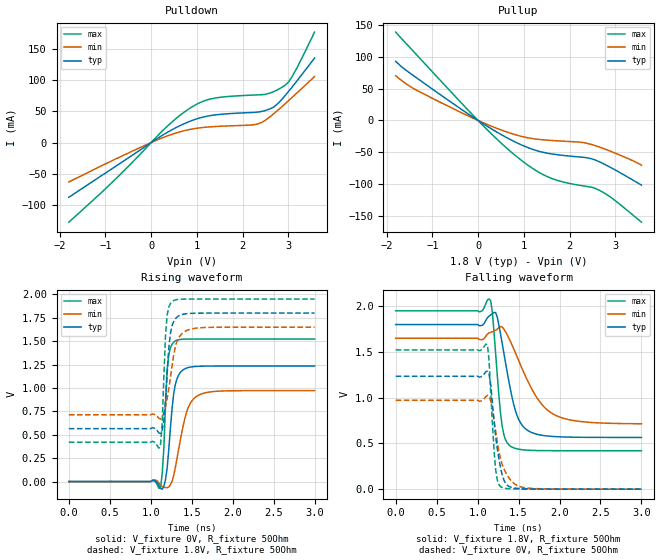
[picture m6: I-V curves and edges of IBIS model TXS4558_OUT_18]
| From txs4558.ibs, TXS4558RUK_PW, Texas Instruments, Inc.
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[Model]   TXS4558_OUT_18
Model_type  Output
Vref =   0
Rref =   50
Cref =   1p
Vmeas =   0.9
| variable   typ   min   max
C_comp   2.08pF   1.15pF   3.73pF
| C_pullup   2.28pF   1.24pF   3.73pF
| C_pulldown   1.87pF   1.15pF   3.52pF
[Temperature Range]   40   100   -40
| Ambient temperature   25   85   -40
[Voltage range]   1.8   1.65   1.95
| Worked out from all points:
|   slope of the pulldown table from 0 to 0.27 V, typ, clamps not added: 21.4 ohm
|   slope of the pullup table from 0 to 0.27 V, typ, clamps not added: 22 ohm
|   falling waveform, V_fixture 1.8V, R_fixture 50Ohm: 20-80 % time 171ps typ, 334ps min, 88.3ps max; typ from 1.8 V to 0.566 V
|   rising waveform, V_fixture 0V, R_fixture 50Ohm: 20-80 % time 79.7ps typ, 143ps min, 47.1ps max; typ from 0 V to 1.24 V
|   rising waveform, V_fixture 1.8V, R_fixture 50Ohm: 20-80 % time 61.8ps typ, 105ps min, 43.8ps max; typ from 0.566 V to 1.8 V
|   falling waveform, V_fixture 0V, R_fixture 50Ohm: 20-80 % time 101ps typ, 138ps min, 61.4ps max; typ from 1.24 V to 0 V
[Pulldown]
| TXS4558_OUT_18
|   Voltage   I(typ)   I(min)   I(max)
-1.8V     -87.61mA   -63.04mA   -127.4mA
-747mV    -36.64mA   -25.32mA   -56.23mA
36mV      1.766mA    1.165mA    2.835mA
468mV     20.94mA    13.46mA    33.68mA
846mV     33.95mA    20.94mA    54.85mA
1.116V    40.38mA    23.96mA    65.37mA
1.386V    44.08mA    25.53mA    71.02mA
2.331V    48.73mA    29.83mA    76.26mA
2.655V    55.79mA    44.55mA    80.69mA
2.925V    74.85mA    61.79mA    91.56mA
3.087V    89.35mA    72.57mA    106.2mA
3.573V    135.2mA    105.6mA    176.7mA
[Pullup]
|   Voltage   I(typ)   I(min)   I(max)
-1.8V     93.31mA    70.46mA    139.4mA
-1.422V   71.22mA    50.78mA    109.7mA
-396mV    19.12mA    13.33mA    30mA
360mV     -16.2mA    -11.02mA   -25.88mA
954mV     -38.76mA   -25.25mA   -63.28mA
1.278V    -47.56mA   -29.5mA    -79.52mA
1.602V    -52.73mA   -31.58mA   -91.25mA
2.277V    -58.02mA   -34.7mA    -103mA
2.493V    -60.7mA    -38.19mA   -105.6mA
2.655V    -65.29mA   -42.01mA   -110.3mA
2.925V    -75.2mA    -49.43mA   -122.4mA
3.573V    -102.1mA   -70.53mA   -160.5mA
[Ramp]
R_load = 50
|   typ   min   max
dV/dt_r   0.740705/7.9653e-11   0.582957/1.42566e-10   0.913773/4.71086e-11
dV/dt_f   0.740477/1.70744e-10   0.560833/3.33892e-10   0.917695/8.83368e-11
[Falling Waveform]
V_fixture = 1.8V
V_fixture_min = 1.65V
V_fixture_max = 1.95V
R_fixture = 50Ohm
C_fixture = 0F
|   Time   V(typ)   V(min)   V(max)
0s        1.8V       1.65V      1.95V
1.02ns    1.788V     1.638V     1.94V
1.16ns    1.905V     1.716V     2.061V
1.22ns    1.931V     1.738V     1.483V
1.3ns     1.593V     1.774V     688.5mV
1.34ns    1.385V     1.723V     542mV
1.42ns    1.007V     1.578V     460mV
1.56ns    681mV      1.283V     429.9mV
1.9ns     577.7mV    833.9mV    421mV
3ns       565.9mV    715.3mV    420.5mV
[Rising Waveform]
V_fixture = 0V
V_fixture_min = 0V
V_fixture_max = 0V
R_fixture = 50Ohm
C_fixture = 0F
|   Time   V(typ)   V(min)   V(max)
0s        2.313nV    13.63nV    255.9pV
1.04ns    13.3mV     16.39mV    7.192mV
1.12ns    -74.43mV   -41.83mV   -62.69mV
1.16ns    -53.55mV   -59.85mV   355.4mV
1.2ns     140.7mV    -65.19mV   1.191V
1.24ns    569.1mV    -36.18mV   1.428V
1.3ns     1.036V     149.4mV    1.503V
1.44ns    1.213V     748.4mV    1.522V
1.58ns    1.231V     921mV      1.523V
3ns       1.235V     971.6mV    1.523V
[Rising Waveform]
V_fixture = 1.8V
V_fixture_min = 1.65V
V_fixture_max = 1.95V
R_fixture = 50Ohm
C_fixture = 0F
|   Time   V(typ)   V(min)   V(max)
0s        565.6mV    713.4mV    420.4mV
1.1ns     519.7mV    675.5mV    356.1mV
1.14ns    550.4mV    688.1mV    625.1mV
1.18ns    868.3mV    797.5mV    1.555V
1.2ns     1.152V     886.4mV    1.779V
1.24ns    1.581V     1.109V     1.902V
1.28ns    1.711V     1.353V     1.934V
1.36ns    1.778V     1.56V      1.948V
1.52ns    1.798V     1.635V     1.95V
3ns       1.8V       1.65V      1.95V
[Falling Waveform]
|Gnd
V_fixture = 0V
V_fixture_min = 0V
V_fixture_max = 0V
R_fixture = 50Ohm
C_fixture = 0F
|   Time   V(typ)   V(min)   V(max)
0s        1.235V     971.8mV    1.523V
1.12ns    1.291V     1.025V     1.577V
1.14ns    1.255V     1.009V     1.402V
1.16ns    1.146V     966.1mV    1.051V
1.22ns    574.6mV    636mV      215.3mV
1.26ns    332mV      410.3mV    49.43mV
1.3ns     156.2mV    269.2mV    17.99mV
1.38ns    31.51mV    127.4mV    5.246mV
1.56ns    4.661mV    18.16mV    1.008mV
3ns       156.9uV    197.2uV    94.19uV
